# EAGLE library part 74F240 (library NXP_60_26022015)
Octal inverting buffer (3-state) The 74F240 is an octal inverting buffer that is ideal for driving bus lines of buffer memory address registers. The outputs are all capable of sinking 64 mA and sourcing up to 15 mA. The device features two output enables, each controlling four of the 3-state outputs. AAL Eindhoven MK
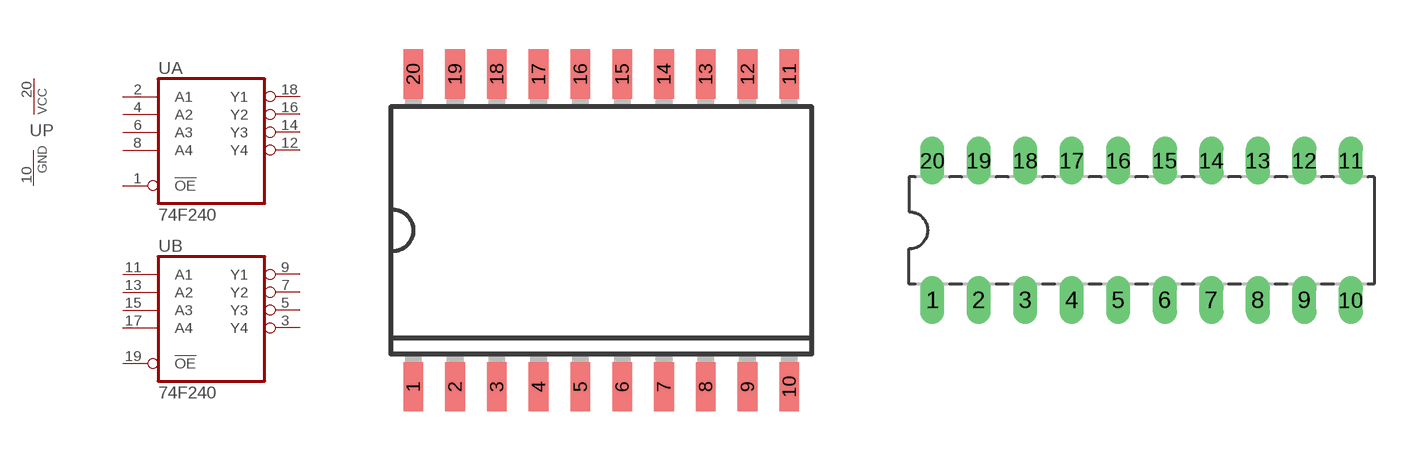
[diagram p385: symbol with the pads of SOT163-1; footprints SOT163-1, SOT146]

Designator prefix U; gates A=74240 B=74240 P=PWRN-3

## 74F240D  [SOT163-1]
1  A:!OE  in
2  A:A1  in
3  B:Y4  hiz
4  A:A2  in
5  B:Y3  hiz
6  A:A3  in
7  B:Y2  hiz
8  A:A4  in
9  B:Y1  hiz
10  P:GND  pwr
11  B:A1  in
12  A:Y4  hiz
13  B:A2  in
14  A:Y3  hiz
15  B:A3  in
16  A:Y2  hiz
17  B:A4  in
18  A:Y1  hiz
19  B:!OE  in
20  P:VCC  pwr

## 74F240N  [SOT146]
Pads as for SOT163-1

## 74F240DB  [SOT339]
Pads as for SOT163-1

## Footprint SOT163-1 (pad centres in mm)
SOT163-1 SO20: plastic small outline package; 20 leads; body width 7.5 mm JEDEC: MS-013 IEC: 075E04
smd 0.6 x 1.5: 1 -5.715,-4.75; 2 -4.445,-4.75; 3 -3.175,-4.75; 4 -1.905,-4.75; 5 -0.635,-4.75; 6 0.635,-4.75; 7 1.905,-4.75; 8 3.175,-4.75; 9 4.445,-4.75; 10 5.715,-4.75; 11 5.715,4.75; 12 4.445,4.75; 13 3.175,4.75; 14 1.905,4.75; 15 0.635,4.75; 16 -0.635,4.75; 17 -1.905,4.75; 18 -3.175,4.75; 19 -4.445,4.75; 20 -5.715,4.75

## Footprint SOT146 (pad centres in mm)
SOT146 DIP20: plastic dual in-line package; 20 leads (300 mil) JEDEC: MS-001 IEC: -- JEITA: SC-603
drill 0.813 long: 1 -11.43,-3.81; 2 -8.89,-3.81; 3 -6.35,-3.81; 4 -3.81,-3.81; 5 -1.27,-3.81; 6 1.27,-3.81; 7 3.81,-3.81; 8 6.35,-3.81; 9 8.89,-3.81; 10 11.43,-3.81; 11 11.43,3.81; 12 8.89,3.81; 13 6.35,3.81; 14 3.81,3.81; 15 1.27,3.81; 16 -1.27,3.81; 17 -3.81,3.81; 18 -6.35,3.81; 19 -8.89,3.81; 20 -11.43,3.81

## Footprint SOT339 (pad centres in mm)
SOT339 SSOP20: plastic shrink small outline package; 20 leads; body width 5.3 mm JEDEC: MO-150 IEC: --
smd 0.4 x 1.1: 1 -2.925,-3.5; 2 -2.275,-3.5; 3 -1.625,-3.5; 4 -0.975,-3.5; 5 -0.325,-3.5; 6 0.325,-3.5; 7 0.975,-3.5; 8 1.625,-3.5; 9 2.275,-3.5; 10 2.925,-3.5; 11 2.925,3.5; 12 2.275,3.5; 13 1.625,3.5; 14 0.975,3.5; 15 0.325,3.5; 16 -0.325,3.5; 17 -0.975,3.5; 18 -1.625,3.5; 19 -2.275,3.5; 20 -2.925,3.5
